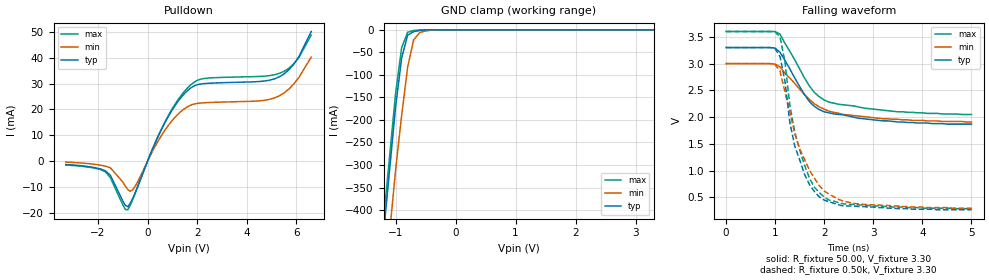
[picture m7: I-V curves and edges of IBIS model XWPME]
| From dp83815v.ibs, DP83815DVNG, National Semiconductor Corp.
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|   Model XWPME
[Model]   XWPME
Model_type   I/O_open_drain
Polarity   Non-Inverting
Enable   Active-High
Vinl =   0.80V
Vinh =   2.00V
Vmeas =   1.50V
Cref =  20.00pF
Rref = 100.00k
C_comp   5.00pF   5.00pF   5.00pF
[Temperature Range]   25.00   0.14k   0.000
[Voltage Range]   3.30V   3.00V   3.60V
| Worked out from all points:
|   slope of the pulldown table from 0 to 0.495 V, typ, clamps not added: 45.1 ohm
|   GND clamp passes 1 mA (typ) near -0.56 V on its own axis
|   falling waveform, R_fixture 50.00, V_fixture 3.30: 20-80 % time 645ps typ, 813ps min, 673ps max; typ from 3.3 V to 1.87 V
|   falling waveform, R_fixture 0.50k, V_fixture 3.30: 20-80 % time 434ps typ, 612ps min, 450ps max; typ from 3.3 V to 0.27 V
[Pulldown]
| voltage   I(typ)   I(min)   I(max)
-3.3V     -1.34mA    -400uA     -1.55mA
-1.7V     -3.79mA    -1.99mA    -4.17mA
-900mV    -17.15mA   -9.69mA    -18.75mA
-800mV    -17.67mA   -11.03mA   -18.86mA
-500mV    -12.32mA   -9.74mA    -12.45mA
600mV     13.04mA    10.54mA    13.23mA
1.2V      22.79mA    17.92mA    23.37mA
1.7V      28.03mA    21.48mA    29.17mA
2.3V      30.02mA    22.6mA     32.01mA
5.3V      32.57mA    25.2mA     33.92mA
5.9V      37.59mA    29.9mA     37.72mA
6.6V      50.19mA    40.25mA    48.83mA
[GND_clamp]
| voltage   I(typ)   I(min)   I(max)
-3.3V     -3.74A     -3.82A     -3.72A
-1.2V     -450mA     -590mA     -420mA
-1.1V     -310mA     -450mA     -280mA
-1V       -170mA     -310mA     -140mA
-900mV    -62.68mA   -190mA     -39.51mA
-800mV    -11.68mA   -82.8mA    -5.29mA
-700mV    -4.09mA    -22.33mA   -1.44mA
-600mV    -1.5mA     -6.16mA    -260uA
-500mV    -290uA     -2.35mA    -23.37uA
-200mV    -65.11nA   -16.16uA   -1.3nA
3.3V      150pA      230nA      35.86pA
[Ramp]
| variable   typ   min   max
dV/dt_r   1.82/2.18n   1.61/2.21n   1.98/2.17n
dV/dt_f   1.82/0.45n   1.62/0.59n   1.98/0.45n
R_load = 0.50k
[Falling Waveform]
R_fixture = 50.00
V_fixture = 3.30
V_fixture_min = 3.00
V_fixture_max = 3.60
| time   V(typ)   V(min)   V(max)
0s        3.3V       3V         3.6V
900ps     3.3V       3V         3.6V
1ns       3.29V      2.99V      3.6V
1.1ns     3.21V      2.94V      3.55V
1.5ns     2.57V      2.52V      2.9V
1.7ns     2.29V      2.33V      2.58V
1.9ns     2.14V      2.19V      2.38V
2.1ns     2.08V      2.11V      2.28V
3.2ns     1.93V      1.97V      2.13V
5ns       1.87V      1.91V      2.05V
[Falling Waveform]
R_fixture = 0.50k
V_fixture = 3.30
V_fixture_min = 3.00
V_fixture_max = 3.60
| time   V(typ)   V(min)   V(max)
0s        3.3V       3V         3.6V
900ps     3.3V       3V         3.6V
1.1ns     3.13V      2.86V      3.5V
1.2ns     2.67V      2.47V      3.03V
1.3ns     1.9V       2.1V       2.22V
1.4ns     1.46V      1.69V      1.72V
1.7ns     740mV      1.01V      860mV
2ns       450mV      620mV      510mV
2.6ns     340mV      390mV      370mV
5ns       270mV      300mV      290mV
